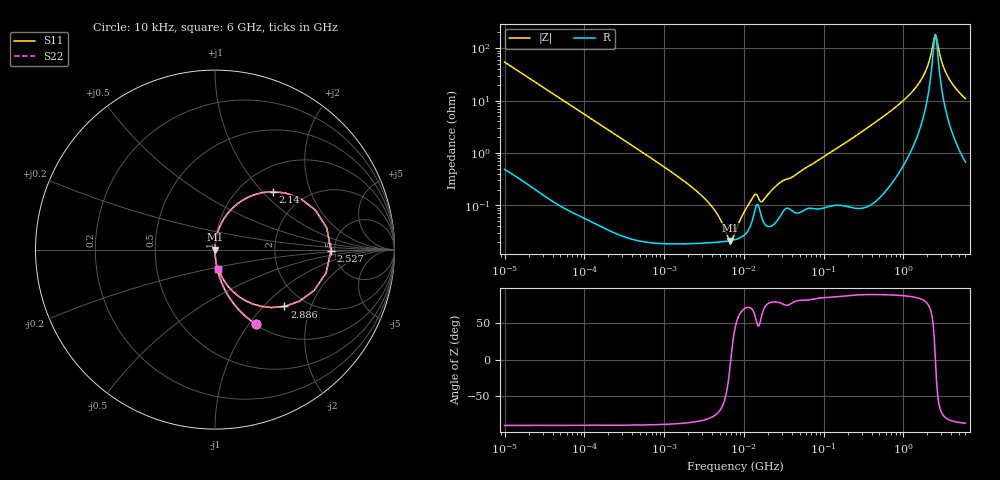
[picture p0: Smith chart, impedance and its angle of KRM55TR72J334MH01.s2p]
!Murata Part Number: KRM55TR72J334MH01
!These Parameters are Measured in Series Mode Connection
!Data Generated on Jan 08, 2026
!  o--ll--o
!Port1  Port2
!  o------o
!Operation Temp=25[degC], DC Bias Voltage=0[V]
!Freq. Start=10[kHz] Stop=6[GHz] 401[Steps]
# Hz S RI R 50
!Freq.(Hz) S11(Real) S11(Imag) S21(Real) S21(Imag) S12(Real) S12(Imag) S22(Real) S22(Imag)
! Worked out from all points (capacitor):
!   401 points, 10 kHz to 6 GHz, reference 50 ohm
!   read as one part in series: C = 293 nF near 10.69 kHz
!   lowest |Z| = 21.2 mohm at 6.781 MHz (marker M1)
!   series resonance near 6.862 MHz, so ESL is about 1.8 nH
!   S11 on the Smith chart (normalised r, x): 10 kHz: 1.01, -1.08; 2.14 GHz: 1.40, +1.15; 2.527 GHz: 4.65, -0.10; 2.886 GHz: 1.58, -1.33; 6 GHz: 1.01, -0.22
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10000  0.229 -0.4158  0.771 0.4158  0.771 0.4158  0.229 -0.4158
23745  0.0517 -0.2171  0.9483 0.2171  0.9483 0.2171  0.0517 -0.2171
92862  0.00406 -0.0587  0.9959 0.0587  0.9959 0.0587  0.00406 -0.0587
862344  0.000227 -0.0063  0.9998 0.0063  0.9998 0.0063  0.000227 -0.0063
3372416  0.000192 -0.00124  0.9998 0.00124  0.9998 0.00124  0.000192 -0.00124
4703216  0.000198 -0.000627  0.9998 0.000627  0.9998 0.000627  0.000198 -0.000627
6781006  0.000211 -1.94e-05  0.9998 1.94e-05  0.9998 1.94e-05  0.000211 -1.94e-05
7745967  0.000221 0.000203  0.9998 -0.000203  0.9998 -0.000203  0.000221 0.000203
9776722  0.00026 0.000628  0.9997 -0.000628  0.9997 -0.000628  0.00026 0.000628
1.363475e7  0.000758 0.00138  0.9992 -0.00138  0.9992 -0.00138  0.000758 0.00138
1.720936e7  0.000526 0.00108  0.9995 -0.00108  0.9995 -0.00108  0.000526 0.00108
2.834297e7  0.000614 0.00263  0.9994 -0.00263  0.9994 -0.00263  0.000614 0.00263
7.193098e7  0.000907 0.00604  0.9991 -0.00604  0.9991 -0.00604  0.000907 0.00604
6.67969e8  0.00587 0.0599  0.9941 -0.0599  0.9941 -0.0599  0.00587 0.0599
1.58612e9  0.0681 0.1981  0.9319 -0.1981  0.9319 -0.1981  0.0681 0.1981
1.873109e9  0.1483 0.2715  0.8517 -0.2715  0.8517 -0.2715  0.1483 0.2715
2.139659e9  0.3219 0.323  0.6781 -0.323  0.6781 -0.323  0.3219 0.323
2.286837e9  0.4765 0.2843  0.5235 -0.2843  0.5235 -0.2843  0.4765 0.2843
2.526803e9  0.6462 -0.00603  0.3538 0.00603  0.3538 0.00603  0.6462 -0.00603
2.886376e9  0.387 -0.3167  0.613 0.3167  0.613 0.3167  0.387 -0.3167
3.643096e9  0.1045 -0.2377  0.8955 0.2377  0.8955 0.2377  0.1045 -0.2377
6e9  0.018 -0.1058  0.982 0.1058  0.982 0.1058  0.018 -0.1058
